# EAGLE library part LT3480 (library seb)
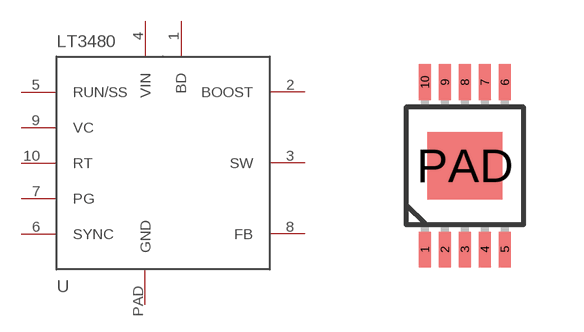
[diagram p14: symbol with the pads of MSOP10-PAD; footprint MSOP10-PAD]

Designator prefix -

## LT3480  [MSOP10-PAD]
1  BD
2  BOOST
3  SW
4  VIN
5  RUN/SS
6  SYNC
7  PG
8  FB
9  VC
10  RT
PAD  GND

## Footprint MSOP10-PAD (pad centres in mm)
smd 0.305 x 0.889: 1 -1,-2.095; 2 -0.5,-2.095; 3 0,-2.095; 4 0.5,-2.095; 5 1,-2.095; 6 1,2.095; 7 0.5,2.095; 8 0,2.095; 9 -0.5,2.095; 10 -1,2.095
smd 1.88 x 1.68: PAD 0,0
